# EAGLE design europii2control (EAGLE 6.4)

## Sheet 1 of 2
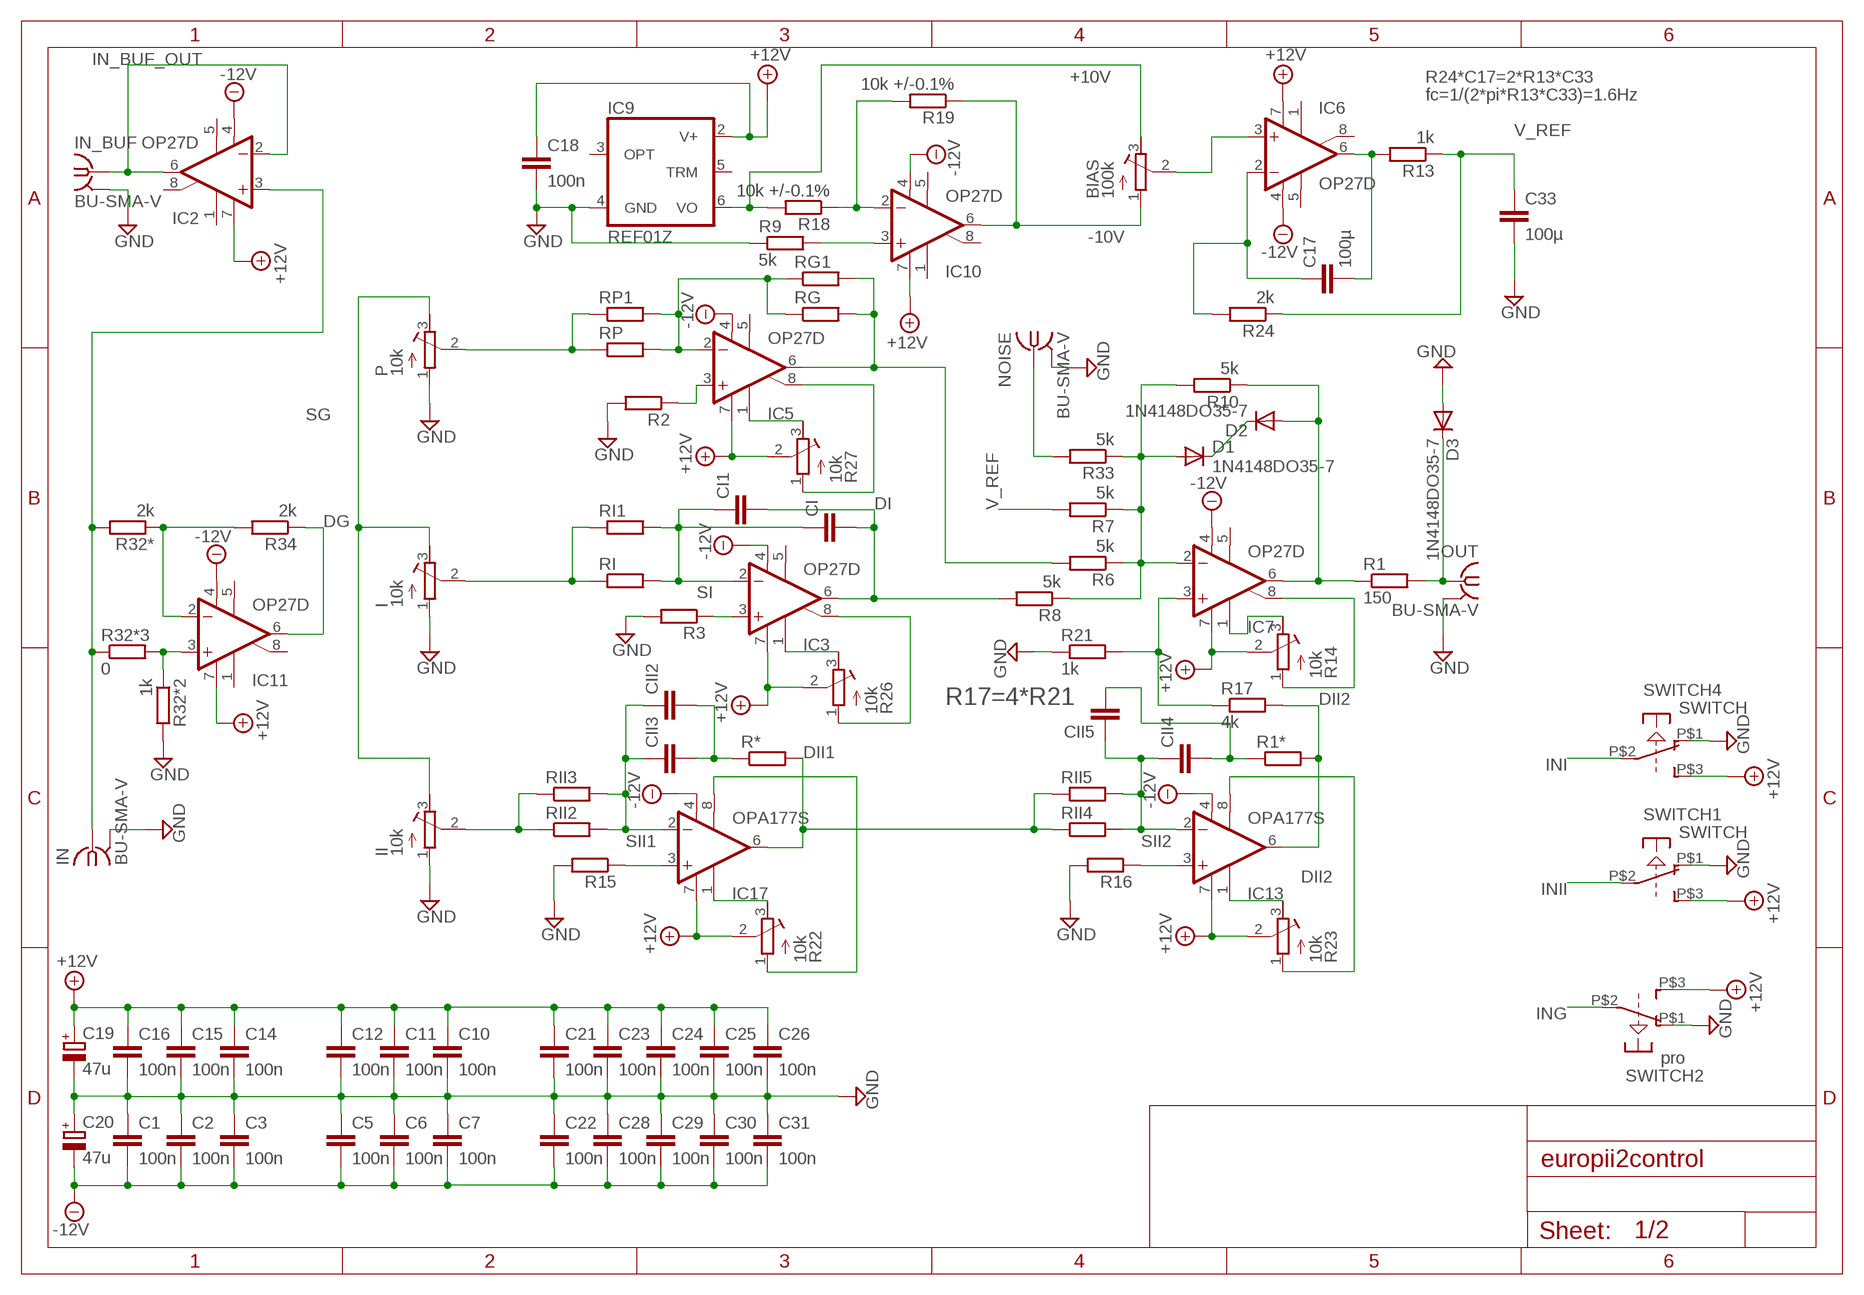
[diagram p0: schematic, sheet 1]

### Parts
BIAS  100k  R-TRIMM64X  [RTRIM64X]
C1  100n  C-EUC0805  [C0805]
C2  100n  C-EUC0805  [C0805]
C3  100n  C-EUC0805  [C0805]
C5  100n  C-EUC0805  [C0805]
C6  100n  C-EUC0805  [C0805]
C7  100n  C-EUC0805  [C0805]
C10  100n  C-EUC0805  [C0805]
C11  100n  C-EUC0805  [C0805]
C12  100n  C-EUC0805  [C0805]
C14  100n  C-EUC0805  [C0805]
C15  100n  C-EUC0805  [C0805]
C16  100n  C-EUC0805  [C0805]
C17  100µ  C-EUC1210K  [C1210K]
C18  100n  C-EUC0805  [C0805]
C19  47u  CPOL-EUCT7343  [CT7343]
C20  47u  CPOL-EUCT7343  [CT7343]
C21  100n  C-EUC0805  [C0805]
C22  100n  C-EUC0805  [C0805]
C23  100n  C-EUC0805  [C0805]
C24  100n  C-EUC0805  [C0805]
C25  100n  C-EUC0805  [C0805]
C26  100n  C-EUC0805  [C0805]
C28  100n  C-EUC0805  [C0805]
C29  100n  C-EUC0805  [C0805]
C30  100n  C-EUC0805  [C0805]
C31  100n  C-EUC0805  [C0805]
C33  100µ  C-EUC1210K  [C1210K]
CI  C-EUC1210  [C1210]
CI1  C-EU050-025X075  [C050-025X075]
CII2  C-EU050-025X075  [C050-025X075]
CII3  C-EUC1210  [C1210]
CII4  C-EUC1210  [C1210]
CII5  C-EU050-025X075  [C050-025X075]
D1  1N4148DO35-7  [DO35-7]
D2  1N4148DO35-7  [DO35-7]
D3  1N4148DO35-7  [DO35-7]
I  10k  R-TRIMM64X  [RTRIM64X]
IC2  OP27D  [SO08]
IC3  OP27D  [SO08]
IC5  OP27D  [SO08]
IC6  OP27D  [SO08]
IC7  OP27D  [SO08]
IC9  REF01Z  [DIL08]
IC10  OP27D  [SO08]
IC11  OP27D  [SO08]
IC13  OPA177S  [SO08]
IC17  OPA177S  [SO08]
II  10k  R-TRIMM64X  [RTRIM64X]
IN  BU-SMA-V  [BU-SMA-V]
IN_BUF  BU-SMA-V  [BU-SMA-V]
NOISE  BU-SMA-V  [BU-SMA-V]
OUT  BU-SMA-V  [BU-SMA-V]
P  10k  R-TRIMM64X  [RTRIM64X]
R1  150  R-EU_R0805  [R0805]
R1*  R-EU_R0805  [R0805]
R2  R-EU_R0805  [R0805]
R3  R-EU_R0805  [R0805]
R6  5k  R-EU_R0805  [R0805]
R7  5k  R-EU_R0805  [R0805]
R8  5k  R-EU_R0805  [R0805]
R9  5k  R-EU_R0805  [R0805]
R10  5k  R-EU_R0805  [R0805]
R13  1k  R-EU_R0805  [R0805]
R14  10k  R-TRIMM3224W  [RTRIM3224W]
R15  R-EU_R0805  [R0805]
R16  R-EU_R0805  [R0805]
R17  4k  R-EU_R0805  [R0805]
R18  10k +/-0.1%  R-EU_R0805  [R0805]
R19  10k +/-0.1%  R-EU_R0805  [R0805]
R21  1k  R-EU_R0805  [R0805]
R22  10k  R-TRIMM3224W  [RTRIM3224W]
R23  10k  R-TRIMM3224W  [RTRIM3224W]
R24  2k  R-EU_R0805  [R0805]
R26  10k  R-TRIMM3224W  [RTRIM3224W]
R27  10k  R-TRIMM3224W  [RTRIM3224W]
R32*  2k  R-EU_R0805  [R0805]
R32*2  1k  R-EU_R0805  [R0805]
R32*3  0  R-EU_R0805  [R0805]
R33  5k  R-EU_R0805  [R0805]
R34  2k  R-EU_R0805  [R0805]
R*  R-EU_R0805  [R0805]
RG  R-EU_R0805  [R0805]
RG1  R-EU_0207/12  [0207/12]
RI  R-EU_R0805  [R0805]
RI1  R-EU_0207/12  [0207/12]
RII2  R-EU_R0805  [R0805]
RII3  R-EU_0207/12  [0207/12]
RII4  R-EU_R0805  [R0805]
RII5  R-EU_0207/12  [0207/12]
RP  R-EU_R0805  [R0805]
RP1  R-EU_0207/12  [0207/12]
SWITCH1  SWITCH  [SWITCH]
SWITCH2  pro  SWITCH  [SWITCH]
SWITCH4  SWITCH  [SWITCH]

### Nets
+10V: BIAS.3(A) IC9.6(VO) R18.2 ; also sheet 2
+12V: C10.1 C11.1 C12.1 C14.1 C15.1 C16.1 C18.1 C19.+ C21.1 C23.1 C24.1 C25.1 C26.1 IC2.7(V+) IC3.7(V+) IC5.7(V+) IC6.7(V+) IC7.7(V+) IC9.2(V+) IC10.7(V+) IC11.7(V+) IC13.7(V+) IC17.7(V+) R14.2(S) R22.2(S) R23.2(S) R26.2(S) R27.2(S) SWITCH1.P$3(S) SWITCH2.P$3(S) SWITCH4.P$3(S) ; also sheet 2
-10V: BIAS.1(E) IC10.6(OUT) R19.1 ; also sheet 2
-12V: C1.2 C2.2 C3.2 C5.2 C6.2 C7.2 C20.- C22.2 C28.2 C29.2 C30.2 C31.2 IC2.4(V-) IC3.4(V-) IC5.4(V-) IC6.4(V-) IC7.4(V-) IC10.4(V-) IC11.4(V-) IC13.4(V-) IC17.4(V-) ; also sheet 2
DG: IC11.6(OUT) R34.1 ; also sheet 2
DI: CI1.2 CI.2 IC3.6(OUT) R8.2 ; also sheet 2
DII1: IC17.6(OUT) R*.2 RII4.1 RII5.1 ; also sheet 2
DII2: IC13.6(OUT) R1*.2 R17.2 ; also sheet 2
ERR_BUF: D2.A IC7.6(OUT) R1.1 R10.1 ; also sheet 2
GND: C1.1 C2.1 C3.1 C5.1 C6.1 C7.1 C10.2 C11.2 C12.2 C14.2 C15.2 C16.2 C18.2 C19.- C20.+ C21.2 C22.1 C23.2 C24.2 C25.2 C26.2 C28.1 C29.1 C30.1 C31.1 C33.2 D3.A I.1(E) IC9.4(GND) II.1(E) IN.2(GND) IN_BUF.2(GND) NOISE.2(GND) OUT.2(GND) P.1(E) R2.2 R3.2 R9.1 R15.2 R16.2 R21.1 R32*2.2 SWITCH1.P$1(O) SWITCH2.P$1(O) SWITCH4.P$1(O) ; also sheet 2
IN_BUF_OUT: IC2.2(-IN) IC2.6(OUT) IN_BUF.1 ; also sheet 2
ING: SWITCH2.P$2(P) ; also sheet 2
INI: SWITCH4.P$2(P) ; also sheet 2
INII: SWITCH1.P$2(P) ; also sheet 2
N$1: IC10.3(+IN) R9.2
N$3: IC3.8(ON2) R26.1(E)
N$4: IC10.2(-IN) R18.1 R19.2
N$5: D1.A IC7.2(-IN) R6.1 R7.1 R8.1 R10.2 R33.1
N$9: IC5.2(-IN) RG1.1 RG.1 RP1.2 RP.2
N$10: IC13.1(TRIM1) R23.3(A)
N$11: II.2(S) RII2.1 RII3.1
N$13: D3.C OUT.1 R1.2
N$15: C17.2 IC6.6(OUT) R13.2
N$17: IC5.3(+IN) R2.1
N$18: IC3.3(+IN) R3.1
N$19: P.2(S) RP1.1 RP.1
N$21: IC11.3(+IN) R32*2.1 R32*3.2
N$24: IC17.3(+IN) R15.1
N$25: IC13.3(+IN) R16.1
N$26: IC7.3(+IN) R17.1 R21.2
N$27: IC7.1(ON1) R14.3(A)
N$28: IC7.8(ON2) R14.1(E)
N$29: IC3.1(ON1) R26.3(A)
N$30: I.2(S) RI1.1 RI.1
N$31: IC17.1(TRIM1) R22.3(A)
N$32: IC5.8(ON2) R27.1(E)
N$33: IC5.1(ON1) R27.3(A)
N$34: IC17.8(TRIM2) R22.1(E)
N$37: IC5.6(OUT) R6.2 RG1.2 RG.2
N$39: D1.C D2.C
N$40: CII2.2 CII3.2 R*.1
N$41: IC11.2(-IN) R32*.1 R34.2
N$42: CII4.2 CII5.2 R1*.1
N$43: IC2.3(+IN) IN.1 R32*3.1 R32*.2
N$46: IC13.8(TRIM2) R23.1(E)
N$47: NOISE.1 R33.2
N$50: C17.1 IC6.2(-IN) R24.2
N$51: BIAS.2(S) IC6.3(+IN)
SG: I.3(A) II.3(A) P.3(A) ; also sheet 2
SI: CI1.1 CI.1 IC3.2(-IN) RI1.2 RI.2 ; also sheet 2
SII1: CII2.1 CII3.1 IC17.2(-IN) RII2.2 RII3.2 ; also sheet 2
SII2: CII4.1 CII5.1 IC13.2(-IN) RII4.2 RII5.2 ; also sheet 2
V_REF: C33.1 R7.2 R13.1 R24.1
Unconnected: IC2.1(ON1) IC2.5(OPT) IC2.8(ON2) IC3.5(OPT) IC5.5(OPT) IC6.1(ON1) IC6.5(OPT) IC6.8(ON2) IC7.5(OPT) IC9.3(OPT) IC9.5(TRM) IC10.1(ON1) IC10.5(OPT) IC10.8(ON2) IC11.1(ON1) IC11.5(OPT) IC11.8(ON2)

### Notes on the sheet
- R24*C17=2*R13*C33
- fc=1/(2*pi*R13*C33)=1.6Hz
- R17=4*R21

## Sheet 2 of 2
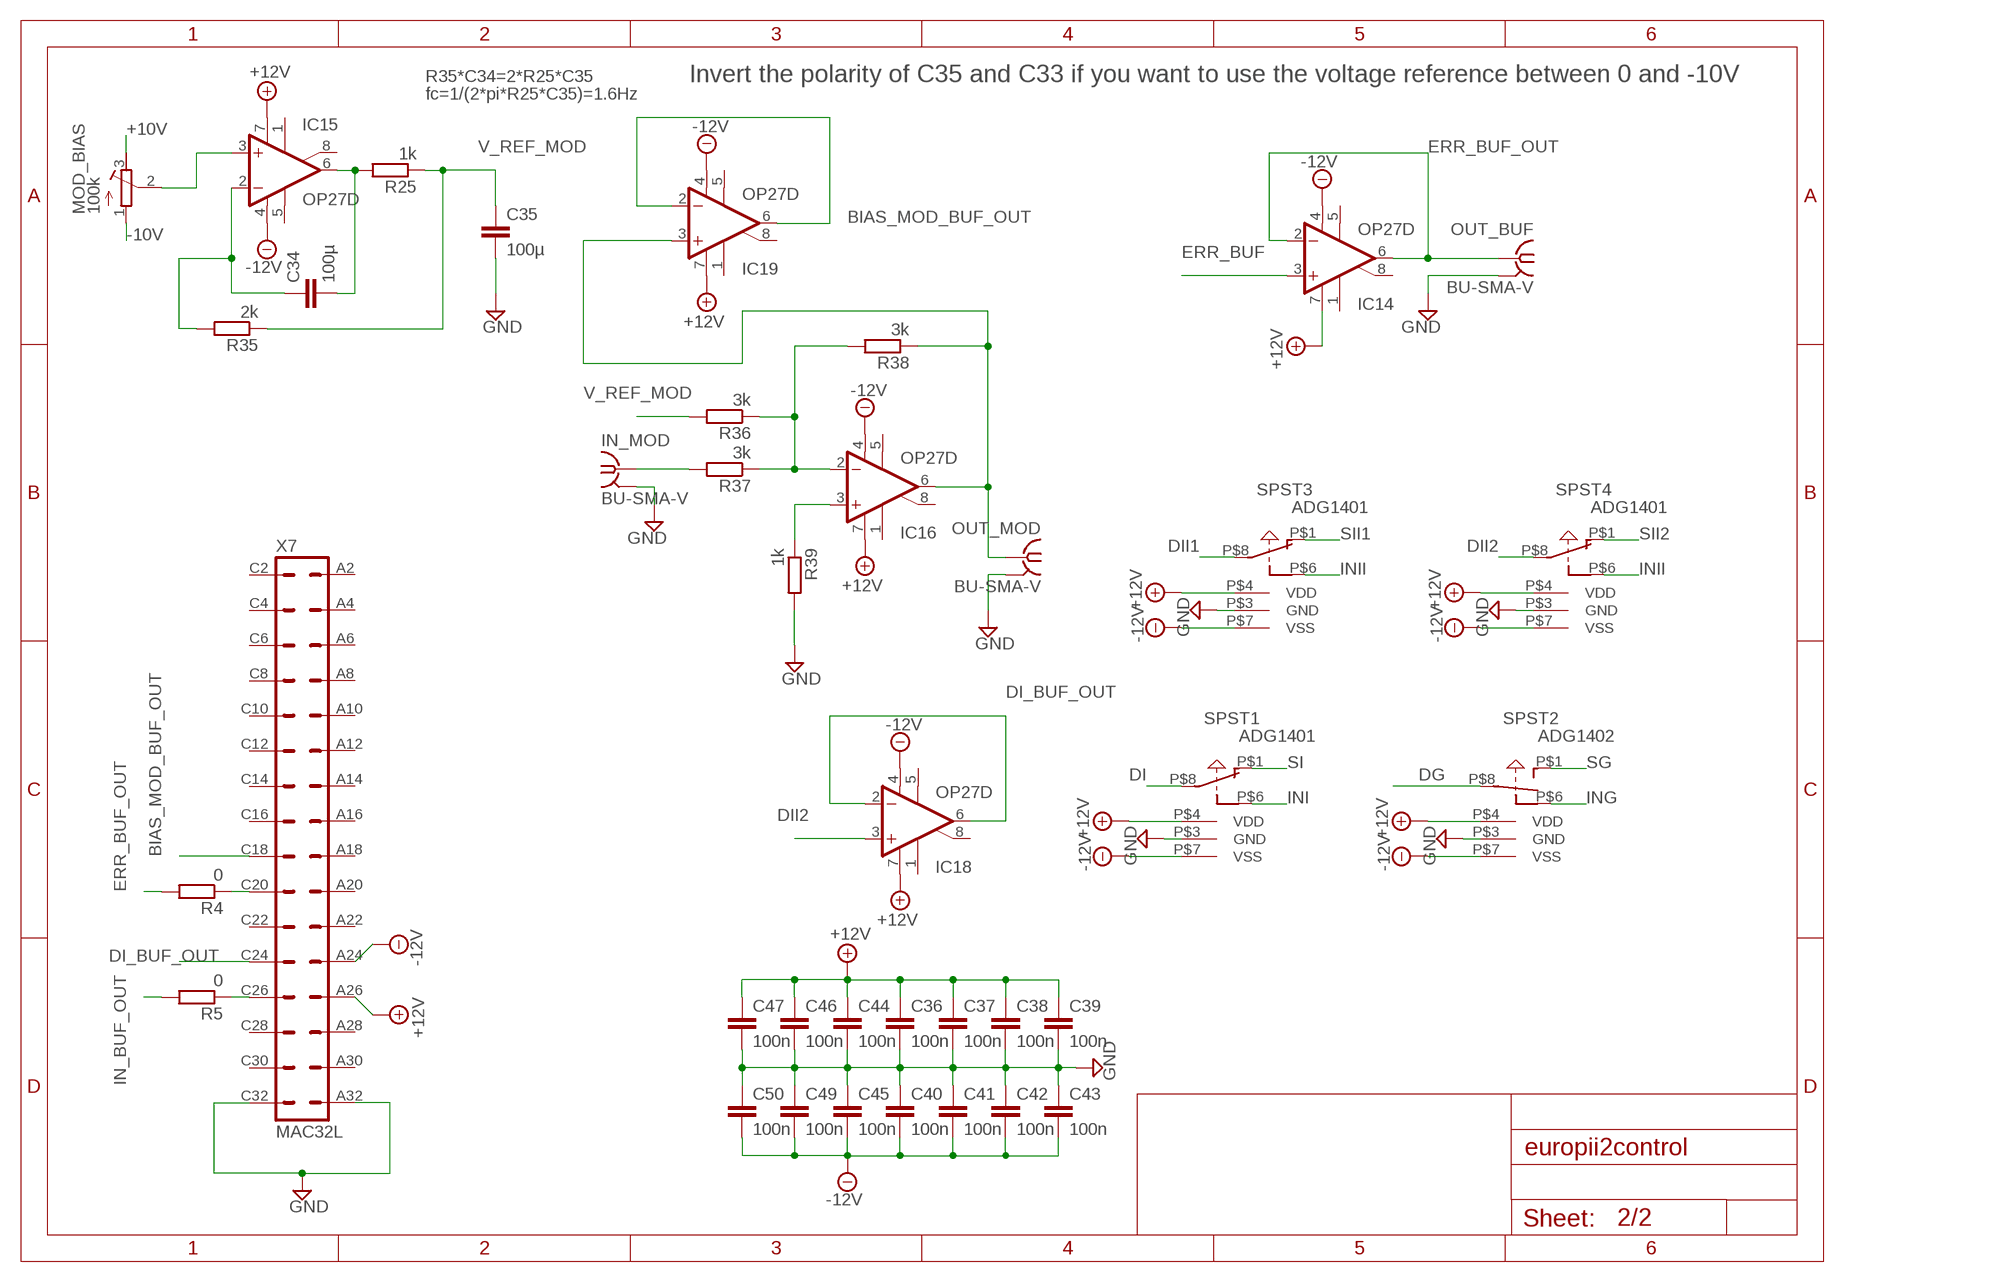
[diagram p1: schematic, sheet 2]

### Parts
C34  100µ  C-EUC1210K  [C1210K]
C35  100µ  C-EUC1210K  [C1210K]
C36  100n  C-EUC0805  [C0805]
C37  100n  C-EUC0805  [C0805]
C38  100n  C-EUC0805  [C0805]
C39  100n  C-EUC0805  [C0805]
C40  100n  C-EUC0805  [C0805]
C41  100n  C-EUC0805  [C0805]
C42  100n  C-EUC0805  [C0805]
C43  100n  C-EUC0805  [C0805]
C44  100n  C-EUC0805  [C0805]
C45  100n  C-EUC0805  [C0805]
C46  100n  C-EUC0805  [C0805]
C47  100n  C-EUC0805  [C0805]
C49  100n  C-EUC0805  [C0805]
C50  100n  C-EUC0805  [C0805]
IC14  OP27D  [SO08]
IC15  OP27D  [SO08]
IC16  OP27D  [SO08]
IC18  OP27D  [SO08]
IC19  OP27D  [SO08]
IN_MOD  BU-SMA-V  [BU-SMA-V]
MOD_BIAS  100k  R-TRIMM64X  [RTRIM64X]
OUT_BUF  BU-SMA-V  [BU-SMA-V]
OUT_MOD  BU-SMA-V  [BU-SMA-V]
R4  0  R-EU_R0805  [R0805]
R5  0  R-EU_R0805  [R0805]
R25  1k  R-EU_R0805  [R0805]
R35  2k  R-EU_R0805  [R0805]
R36  3k  R-EU_R0805  [R0805]
R37  3k  R-EU_R0805  [R0805]
R38  3k  R-EU_R0805  [R0805]
R39  1k  R-EU_R0805  [R0805]
SPST1  ADG1401  [MSOP-RM8]
SPST2  ADG1402  [MSOP-RM8]
SPST3  ADG1401  [MSOP-RM8]
SPST4  ADG1401  [MSOP-RM8]
X7  MAC32L  [MAC32L]

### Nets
+10V: MOD_BIAS.3(A) ; also sheet 1
+12V: C36.1 C37.1 C38.1 C39.1 C44.1 C46.1 C47.1 IC14.7(V+) IC15.7(V+) IC16.7(V+) IC18.7(V+) IC19.7(V+) SPST1.P$4(VDD) SPST2.P$4(VDD) SPST3.P$4(VDD) SPST4.P$4(VDD) X7.A26 ; also sheet 1
-10V: MOD_BIAS.1(E) ; also sheet 1
-12V: C40.2 C41.2 C42.2 C43.2 C45.2 C49.2 C50.2 IC14.4(V-) IC15.4(V-) IC16.4(V-) IC18.4(V-) IC19.4(V-) SPST1.P$7(VSS) SPST2.P$7(VSS) SPST3.P$7(VSS) SPST4.P$7(VSS) X7.A24 ; also sheet 1
BIAS_MOD_BUF_OUT: IC19.2(-IN) IC19.6(OUT) X7.C18
DG: SPST2.P$8(D) ; also sheet 1
DI: SPST1.P$8(D) ; also sheet 1
DI_BUF_OUT: IC18.2(-IN) IC18.6(OUT) X7.C24
DII1: SPST3.P$8(D) ; also sheet 1
DII2: IC18.3(+IN) SPST4.P$8(D) ; also sheet 1
ERR_BUF: IC14.3(+IN) ; also sheet 1
ERR_BUF_OUT: IC14.2(-IN) IC14.6(OUT) OUT_BUF.1 R4.2
GND: C35.2 C36.2 C37.2 C38.2 C39.2 C40.1 C41.1 C42.1 C43.1 C44.2 C45.1 C46.2 C47.2 C49.1 C50.1 IN_MOD.2(GND) OUT_BUF.2(GND) OUT_MOD.2(GND) R39.2 SPST1.P$3(GND) SPST2.P$3(GND) SPST3.P$3(GND) SPST4.P$3(GND) X7.A32 X7.C32 ; also sheet 1
IN_BUF_OUT: R5.2 ; also sheet 1
ING: SPST2.P$6(IN) ; also sheet 1
INI: SPST1.P$6(IN) ; also sheet 1
INII: SPST3.P$6(IN) SPST4.P$6(IN) ; also sheet 1
N$6: R4.1 X7.C20
N$7: IC16.3(+IN) R39.1
N$8: IN_MOD.1 R37.2
N$16: IC16.2(-IN) R36.1 R37.1 R38.2
N$20: IC16.6(OUT) IC19.3(+IN) OUT_MOD.1 R38.1
N$38: R5.1 X7.C26
N$52: C34.2 IC15.6(OUT) R25.2
N$53: C34.1 IC15.2(-IN) R35.2
N$54: IC15.3(+IN) MOD_BIAS.2(S)
SG: SPST2.P$1(S) ; also sheet 1
SI: SPST1.P$1(S) ; also sheet 1
SII1: SPST3.P$1(S) ; also sheet 1
SII2: SPST4.P$1(S) ; also sheet 1
V_REF_MOD: C35.1 R25.1 R35.1 R36.2
Unconnected: IC14.1(ON1) IC14.5(OPT) IC14.8(ON2) IC15.1(ON1) IC15.5(OPT) IC15.8(ON2) IC16.1(ON1) IC16.5(OPT) IC16.8(ON2) IC18.1(ON1) IC18.5(OPT) IC18.8(ON2) IC19.1(ON1) IC19.5(OPT) IC19.8(ON2) X7.A2 X7.A4 X7.A6 X7.A8 X7.A10 X7.A12 X7.A14 X7.A16 X7.A18 X7.A20 X7.A22 X7.A28 X7.A30 X7.C2 X7.C4 X7.C6 X7.C8 X7.C10 X7.C12 X7.C14 X7.C16 X7.C22 X7.C28 X7.C30

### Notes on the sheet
- R35*C34=2*R25*C35 | Invert the polarity of C35 and C33 if you want to use the voltage reference between 0 and -10V
- fc=1/(2*pi*R25*C35)=1.6Hz

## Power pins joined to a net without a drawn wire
GND: IN.3(GND) IN.4(GND) IN.5(GND) IN_BUF.3(GND) IN_BUF.4(GND) IN_BUF.5(GND) IN_MOD.3(GND) IN_MOD.4(GND) IN_MOD.5(GND) NOISE.3(GND) NOISE.4(GND) NOISE.5(GND) OUT.3(GND) OUT.4(GND) OUT.5(GND) OUT_BUF.3(GND) OUT_BUF.4(GND) OUT_BUF.5(GND) OUT_MOD.3(GND) OUT_MOD.4(GND) OUT_MOD.5(GND)

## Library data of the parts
BIAS I II MOD_BIAS P R14 R22 R23 R26 R27 = rcl:R-TRIMM: Trimm resistor
C1-C3 C5-C7 C10-C12 C14-C18 C21-C26 C28-C31 C33-C47 C49 C50 CI CI1 CII2-CII5 = rcl:C-EU: CAPACITOR, European symbol
C19 C20 = rcl:CPOL-EU: POLARIZED CAPACITOR, European symbol
D1-D3 = diode:1N4148: DIODE
IC2 IC3 IC5-IC7 IC10 IC11 IC14-IC16 IC18 IC19 = linear:OP27: OP AMP
IC9 = linear:REF01: VOLTAGE REFERENCE
IC13 IC17 = burr-brown:OPA177: Precision Operational Amplifier
IN IN_BUF IN_MOD NOISE OUT OUT_BUF OUT_MOD = con-coax:BU-SMA-V: FEMALE SMA CONNECTOR Radiall distributor RS 112-3794
R1 R1* R2-R10 R13 R15-R19 R21 R24 R25 R32* R32*2 R32*3 R33-R39 R* RG RG1 RI RI1 RII2-RII5 RP RP1 = rcl:R-EU_: RESISTOR, European symbol
SPST1 SPST3 SPST4 = srinos-lib:ADG1401
SPST2 = srinos-lib:ADG1402
SWITCH1 SWITCH2 SWITCH4 = srinos-lib:SWITCH
X7 = con-vg:MAC32L: CONNECTOR male, 32 pins, block, type D, rows AC, grid 5.08 mm with mounting clip

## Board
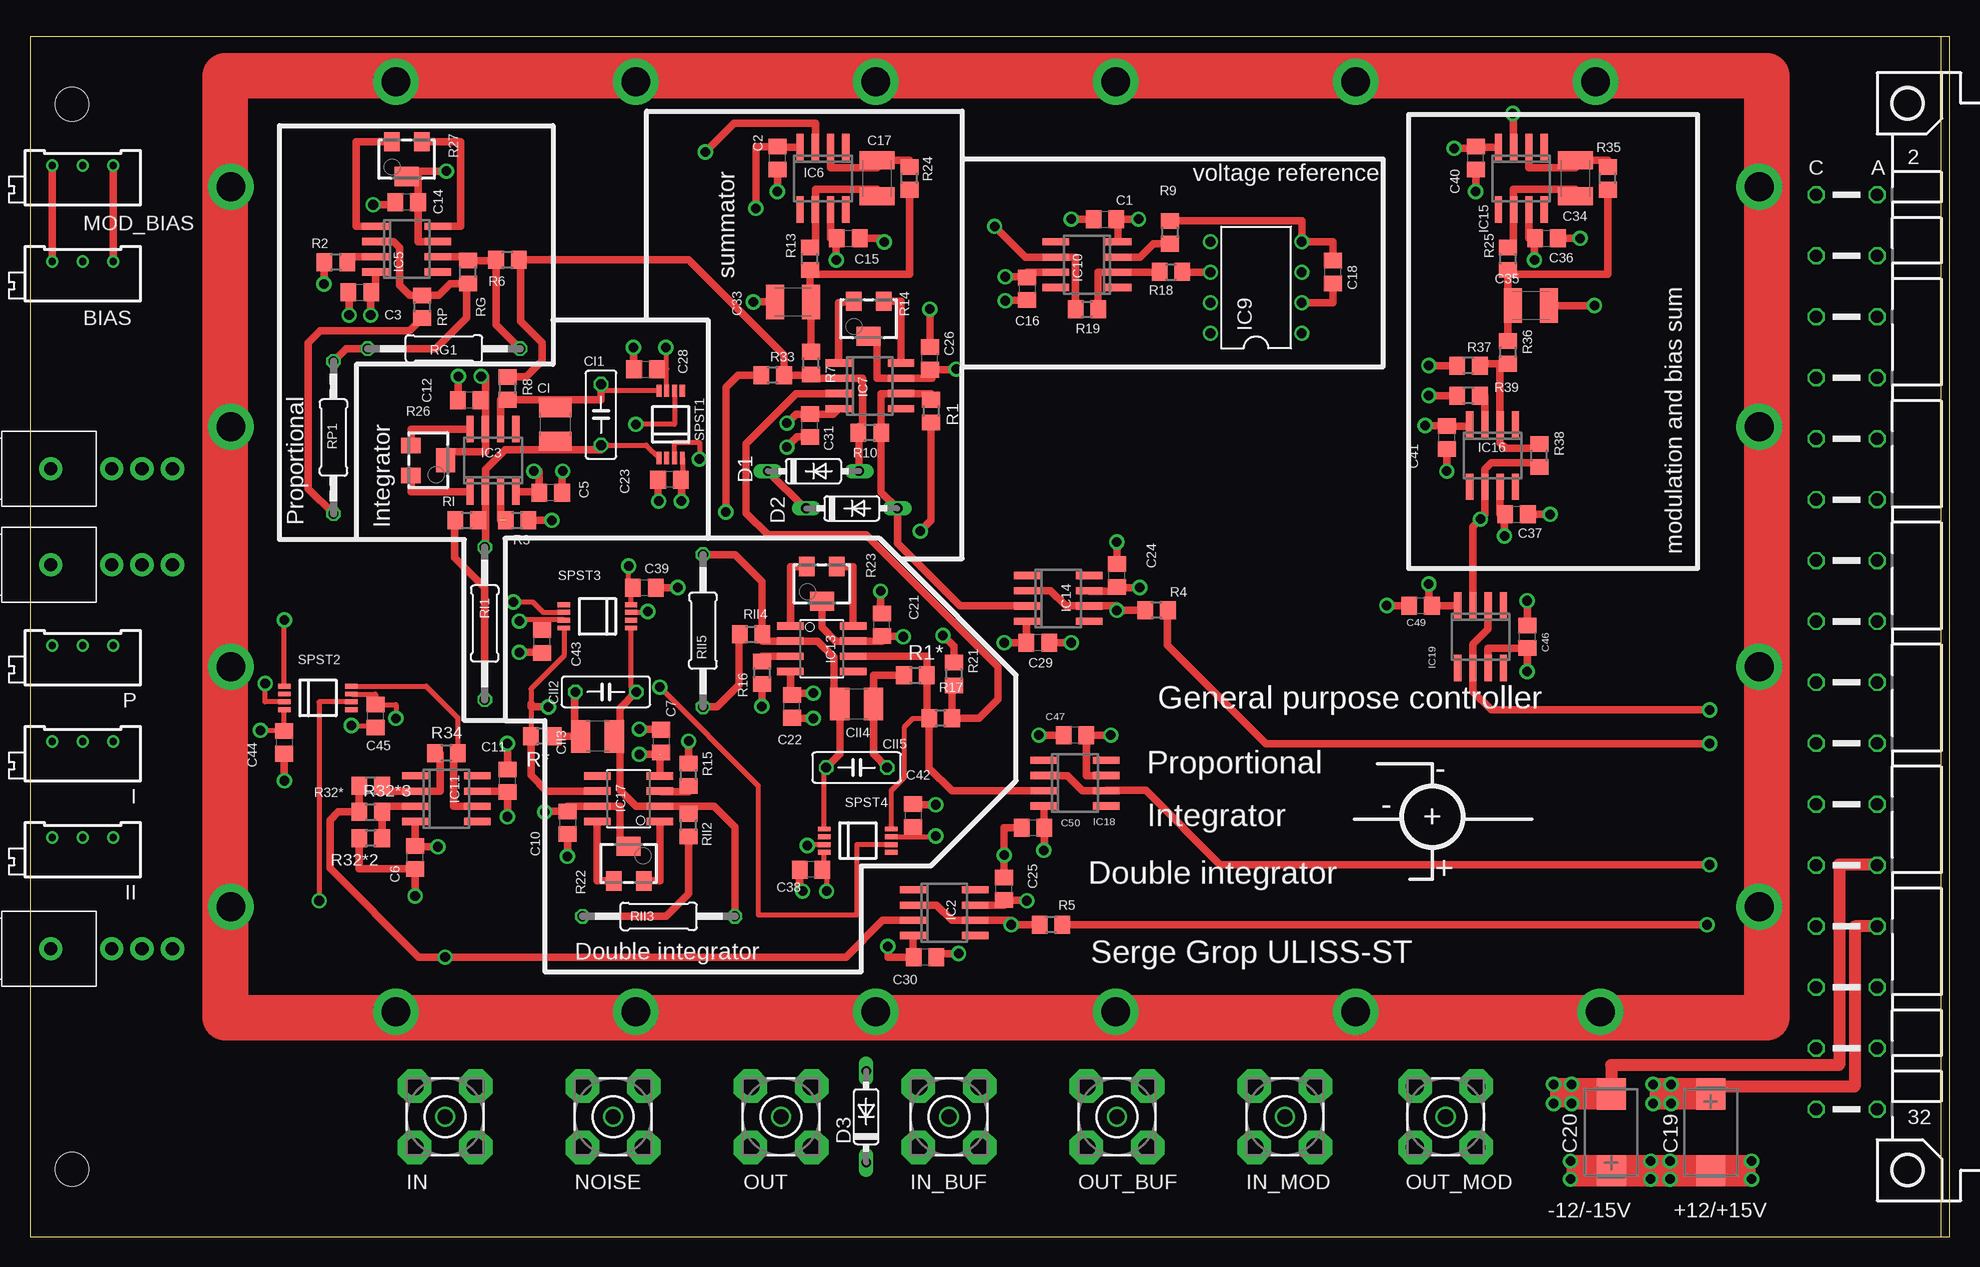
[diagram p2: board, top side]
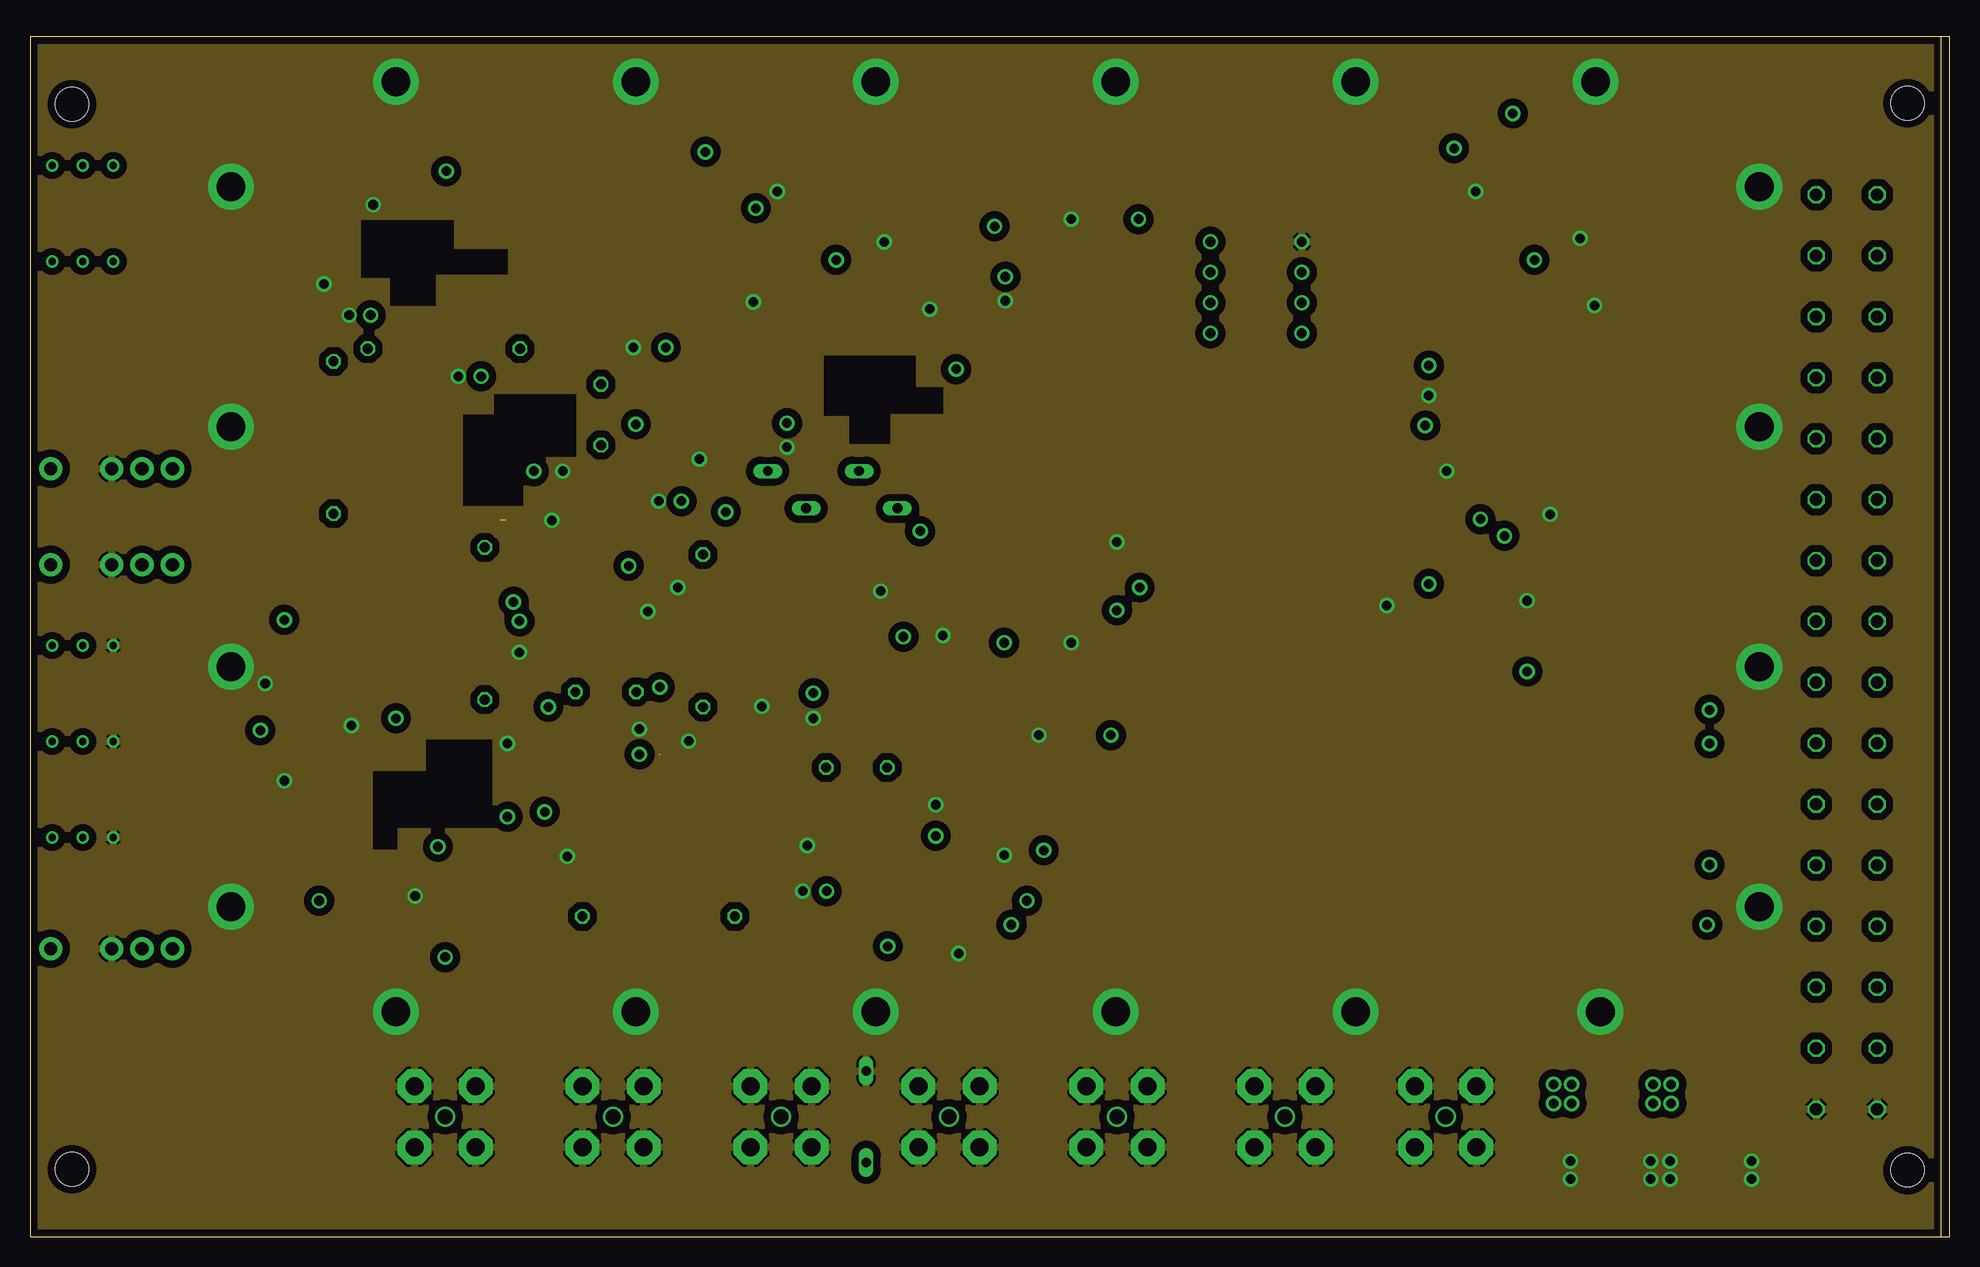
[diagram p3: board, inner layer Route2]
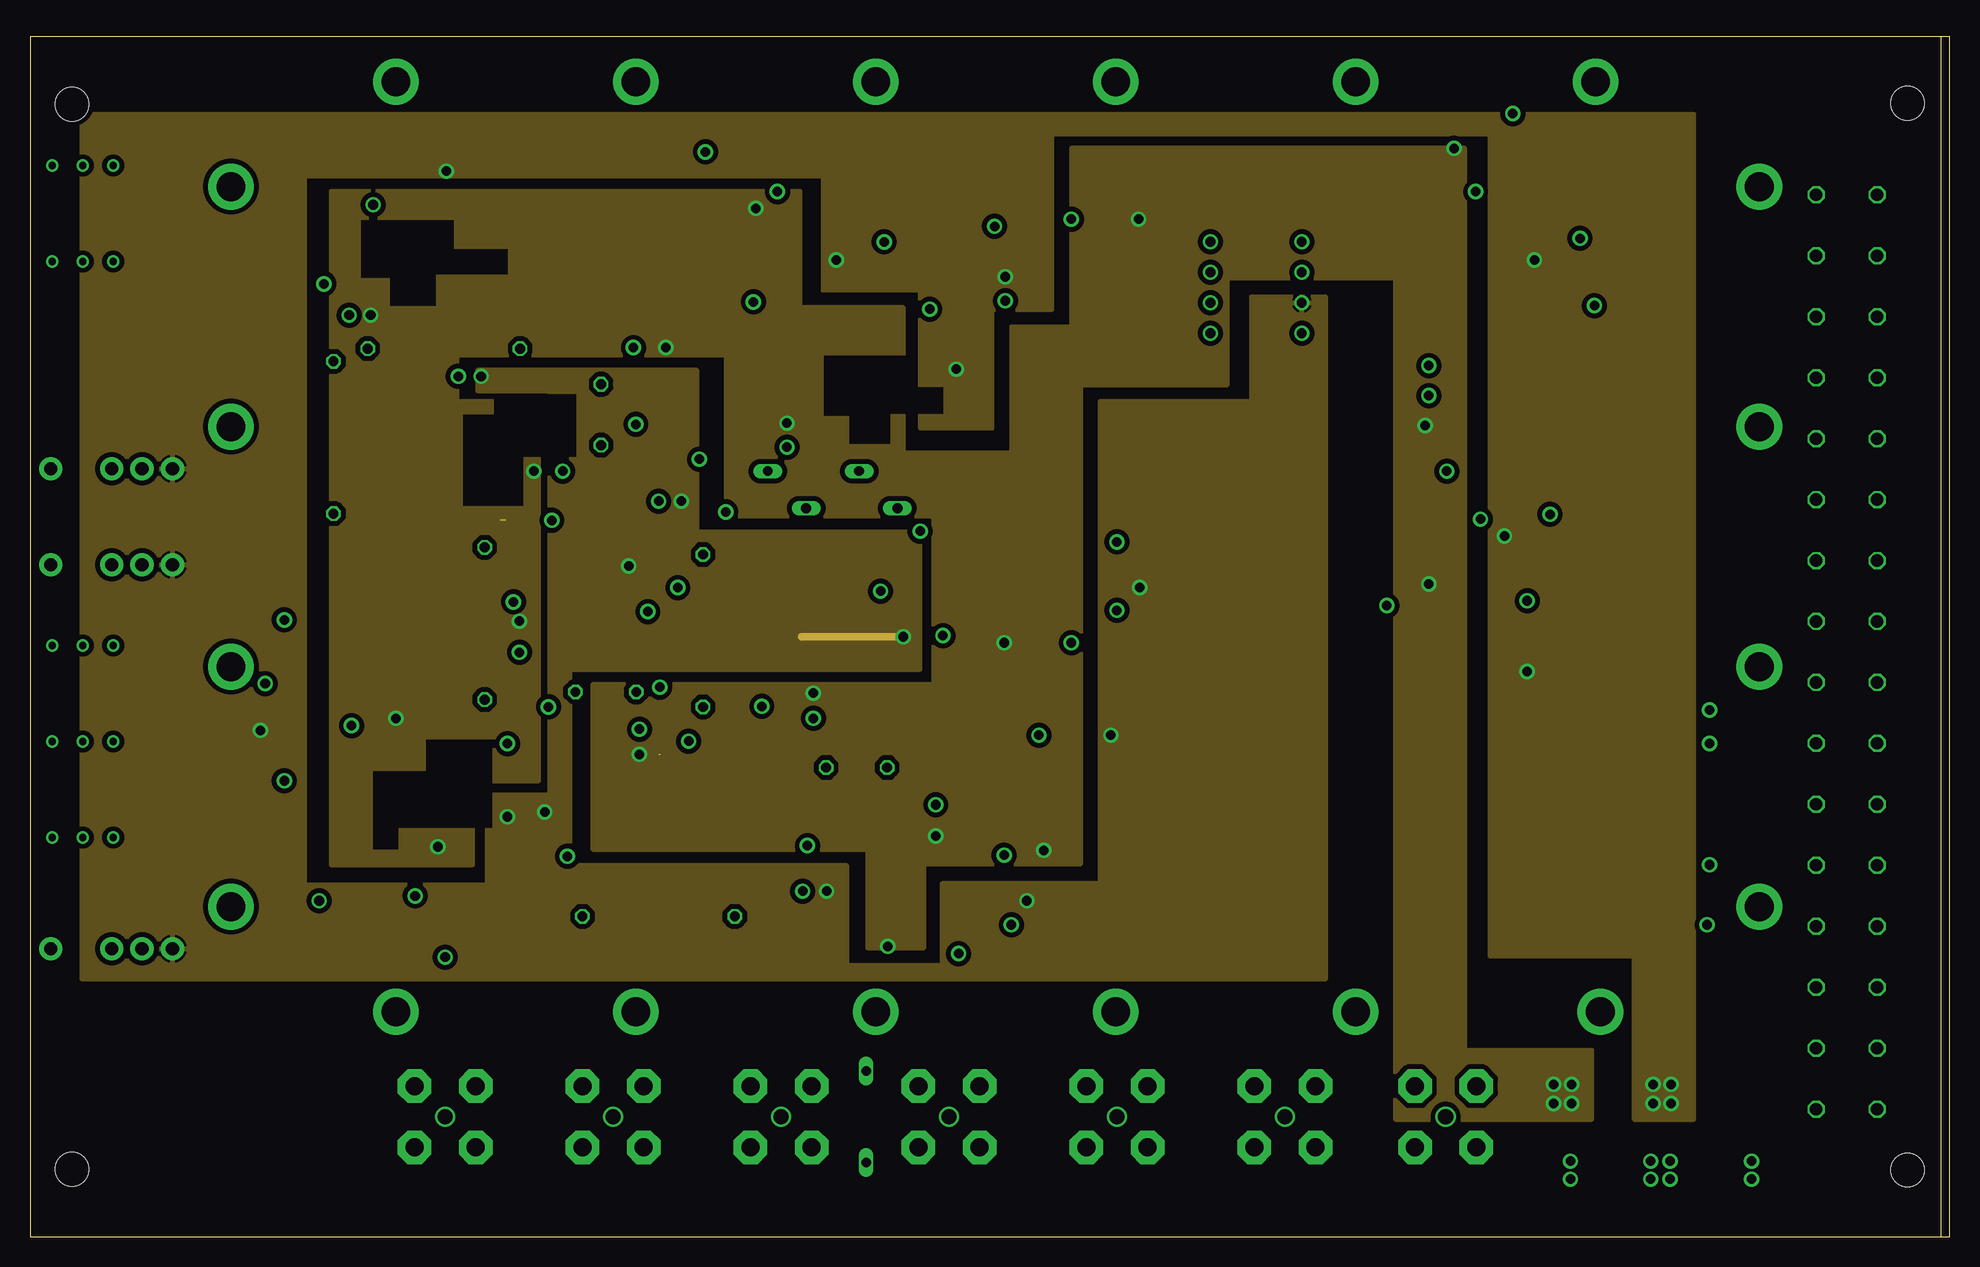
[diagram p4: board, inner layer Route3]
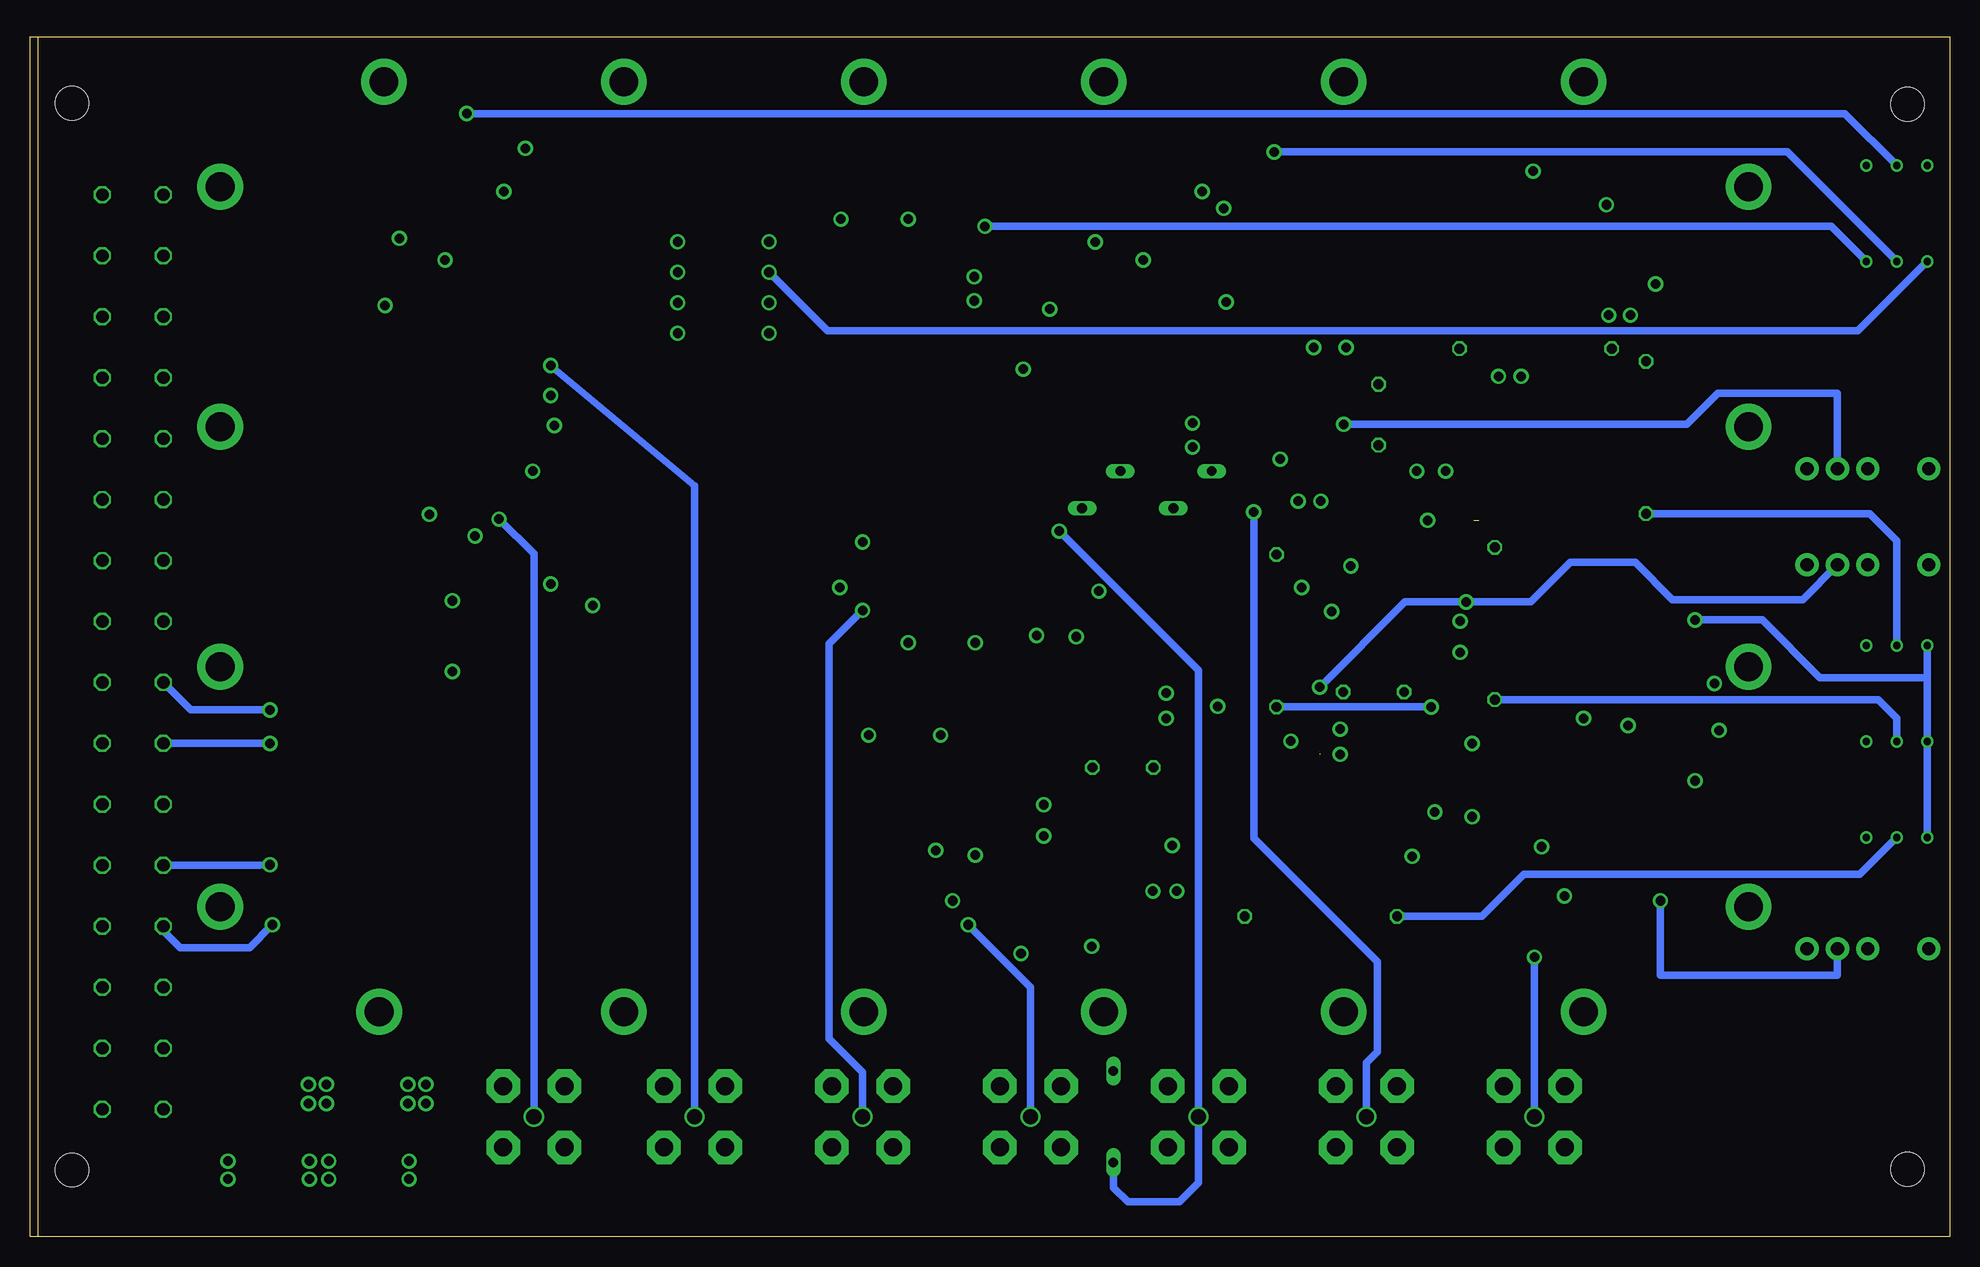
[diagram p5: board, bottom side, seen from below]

Size 160 x 100.03 mm. Coordinates in mm from the lower left corner, seen from the top.
Outline: 0,0.01 160,0.01 160,100.01 0,100.01 0,0.01
Copper layers (1*2*3*16): Top 0.035mm / dielectric 0.38mm / Route2 0.035mm / dielectric 0.71mm / Route3 0.035mm / dielectric 0.38mm / Bottom 0.035mm
Design rules "PCB-POOL-Standard-4-layers": minimum track width 0.15mm, minimum drill 0.3mm, track to track 0.15mm, track to pad 0.15mm, pad to pad 0.15mm, via to via 0.15mm, smd to smd 0.15mm, copper to edge 0.3mm, drill to drill 0.2mm, minimum pad ring 0.2mm, minimum via ring 0.15mm, stop-mask expansion 0.075mm, vias tented up to drill 0mil, thermal gap 0.2mm
Holes 2.8 mm at 3.5,5.64 3.5,94.39

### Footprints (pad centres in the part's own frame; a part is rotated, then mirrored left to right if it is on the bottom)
RTRIM64X = drill 0.61: 1 1.27,-2.54; 2 1.27,0; 3 1.27,2.54
C0805 = smd 1.3 x 1.5: 1 -0.95,0; 2 0.95,0
C1210K = smd 1.5 x 2.9: 1 -1.5,0; 2 1.5,0
CT7343 = smd 2.6 x 2.4: + -3.2,0; - 3.2,0
C1210 = smd 1.6 x 2.7: 1 -1.4,0; 2 1.4,0
C050-025X075 = drill 0.813 octagon: 1 -2.54,0; 2 2.54,0
DO35-7 = drill 0.813 long: A 3.81,0; C -3.81,0
SO08 = smd 0.6 x 2.2: 1 -1.905,-2.6; 2 -0.635,-2.6; 3 0.635,-2.6; 4 1.905,-2.6; 5 1.905,2.6; 6 0.635,2.6; 7 -0.635,2.6; 8 -1.905,2.6
DIL08 = drill 0.813 pad 1.27: 1 -3.81,-3.81; 2 -1.27,-3.81; 3 1.27,-3.81; 4 3.81,-3.81; 5 3.81,3.81; 6 1.27,3.81; 7 -1.27,3.81; 8 -3.81,3.81
SO08' = smd 0.61 x 2.21: 1 -1.905,-2.616; 2 -0.635,-2.616; 3 0.635,-2.616; 4 1.905,-2.616; 5 1.905,2.616; 6 0.635,2.616; 7 -0.635,2.616; 8 -1.905,2.616
BU-SMA-V = drill 1.27: 1 0,0 | drill 1.5 pad 2.794 octagon: 2 -2.55,2.55; 3 2.55,2.55; 4 2.55,-2.55; 5 -2.55,-2.55
R0805 = smd 1.3 x 1.5: 1 -0.95,0; 2 0.95,0
RTRIM3224W = smd 1.3 x 1.6: 1 -1.25,-1.45; 3 1.25,-1.45 | smd 2 x 1.6: 2 0,1.45
0207/12 = drill 0.813 octagon: 1 -6.35,0; 2 6.35,0
MSOP-RM8 = smd 0.41 x 1.02: P$1 -0.975,-2.8; P$2 -0.325,-2.8; P$3 0.325,-2.8; P$4 0.975,-2.8; P$6 0.325,2.8; P$7 -0.325,2.8; P$8 -0.975,2.8 | smd 0.42 x 1.02: P$5 0.975,2.8
SWITCH = drill 1.1 pad 1.93: P$1 0,0; P$2 0,2.54; P$3 0,5.08; P$4 0,-5.08
MAC32L = drill 1.016 octagon: A2 -2.54,36.83; A4 -2.54,31.75; A6 -2.54,26.67; A8 -2.54,21.59; A10 -2.54,16.51; A12 -2.54,11.43; A14 -2.54,6.35; A16 -2.54,1.27; A18 -2.54,-3.81; A20 -2.54,-8.89; A22 -2.54,-13.97; A24 -2.54,-19.05; A26 -2.54,-24.13; A28 -2.54,-29.21; A30 -2.54,-34.29; A32 -2.54,-39.37; C2 -7.62,36.83; C4 -7.62,31.75; C6 -7.62,26.67; C8 -7.62,21.59; C10 -7.62,16.51; C12 -7.62,11.43; C14 -7.62,6.35; C16 -7.62,1.27; C18 -7.62,-3.81; C20 -7.62,-8.89; C22 -7.62,-13.97; C24 -7.62,-19.05; C26 -7.62,-24.13; C28 -7.62,-29.21; C30 -7.62,-34.29; C32 -7.62,-39.37 | hole 2.794: 0,44.45; 0,-44.45

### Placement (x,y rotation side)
BIAS  4.4,80.01 90 top
C1  89.6,84.81 0 top
C2  62.3,89.91 90 top
C3  27.5,78.71 0 top
C5  43.4,62.01 180 top
C6  32.1,31.61 90 top
C7  52.6,41.31 270 top
C10  44.8,34.51 270 top
C11  39.8,38.01 90 top
C12  36.6,69.71 180 top
C14  31.4,86.21 180 top
C15  68.2,83.21 0 top
C16  83.1,79.01 270 top
C17  70.6,88.21 270 top
C18  108.6,80.41 90 top
C19  140.1,8.71 270 top
C20  131.8,8.71 90 top
C21  71,51.01 90 top
C22  63.5,44.21 90 top
C23  53.3,63.11 180 top
C24  90.6,55.11 90 top
C25  81.2,29.01 90 top
C26  75,73.21 90 top
C28  51.3,72.31 0 top
C29  84,49.51 180 top
C30  74.6,23.31 180 top
C31  65,67.61 90 top
C33  63.6,77.91 180 top
C34  128.8,88.21 270 top
C35  125.1,77.61 0 top
C36  126.4,83.21 0 top
C37  123.9,60.21 0 top
C38  65.1,30.61 180 top
C39  51.2,54.11 0 top
C40  120.5,89.91 90 top
C41  118.1,66.61 90 top
C42  73.6,35.11 270 top
C43  42.7,49.61 90 top
C44  21.2,41.21 270 top
C45  28.8,43.41 90 top
C46  124.8,50.01 90 top
C47  87.1,41.81 180 top
C49  115.9,52.61 0 top
C50  83.6,34.11 0 top
CI  43.8,67.71 90 top
CI1  47.6,68.51 90 top
CII2  48,45.41 180 top
CII3  47.3,41.71 180 top
CII4  68.9,44.41 0 top
CII5  68.9,39.11 0 top
D1  65.3,63.81 0 top
D2  68.5,60.71 0 top
D3  69.7,10.01 90 top
I  4.4,40.01 90 top
IC2  76.2,27.01 270 top
IC3  38.6,64.71 0 top
IC5  31.4,82.31 270 top
IC6  66.1,88.21 180 top
IC7  70,70.91 270 top
IC9  102.2,79.11 90 top
IC10  88.1,81.01 90 top
IC11  34.7,36.51 270 top
IC13  OPA177S  [SO08']  66,49.01 270 top
IC14  85.7,53.21 270 top
IC15  124.3,88.21 180 top
IC16  121.9,65.11 180 top
IC17  OPA177S  [SO08']  49.9,36.51 90 top
IC18  87.1,37.81 270 top
IC19  120.9,50.01 180 top
II  4.4,32.01 90 top
IN  34.6,10.01 0 top
IN_BUF  76.6,10.01 0 top
IN_MOD  104.6,10.01 0 top
MOD_BIAS  4.4,88.01 90 top
NOISE  48.6,10.01 0 top
OUT  62.6,10.01 0 top
OUT_BUF  90.6,10.01 0 top
OUT_MOD  118,10.01 0 top
P  4.4,48.01 90 top
R1  75.1,68.81 270 top
R1*  73.8,46.81 0 top
R2  25.5,81.21 180 top
R3  40.6,59.71 0 top
R4  93.9,52.21 180 top
R5  85.1,26.01 180 top
R6  39.8,81.41 180 top
R7  65.1,72.81 90 top
R8  39.8,70.71 270 top
R9  95,83.71 270 top
R10  70,67.01 180 top
R13  65,81.51 90 top
R14  69.9,76.51 180 top
R15  54.9,38.51 90 top
R16  61,47.01 270 top
R17  75.9,43.21 180 top
R18  95.1,80.41 0 top
R19  88.1,77.31 0 top
R21  77,46.91 270 top
R22  49.9,31.11 0 top
R23  66,54.41 180 top
R24  73.3,88.21 90 top
R25  123.2,81.51 90 top
R26  33.2,64.71 270 top
R27  31.4,89.81 180 top
R32*  28.4,37.61 180 top
R32*2  28.4,33.21 180 top
R32*3  28.4,35.41 0 top
R33  61.9,71.81 180 top
R34  34.7,40.31 180 top
R35  131.5,88.21 90 top
R36  123.2,73.71 90 top
R37  119.9,72.61 180 top
R38  125.8,65.11 90 top
R39  119.9,70.11 180 top
R*  42.7,41.71 180 top
RG  36.5,80.41 90 top
RG1  34.5,74.01 0 top
RI  36.4,59.71 0 top
RI1  37.9,51.11 90 top
RII2  54.9,34.31 90 top
RII3  52.4,26.71 0 top
RII4  60.1,50.21 0 top
RII5  56.1,50.51 90 top
RP  32.7,77.51 90 top
RP1  25.3,66.61 90 top
SPST1  53.4,67.71 0 top
SPST2  24,44.91 270 top
SPST3  47.3,51.71 90 top
SPST4  69,33.01 270 top
SWITCH1  6.8,56.01 270 top
SWITCH2  6.8,24.01 270 top
SWITCH4  6.8,64.01 270 top
X7  156.5,50.01 0 top

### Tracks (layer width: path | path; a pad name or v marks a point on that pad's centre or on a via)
+10V
  Top 0.61: IC9.6 96.05,80.38 R18.2 | BIAS.3 MOD_BIAS.3
  Bottom 0.61: IC9.6 93.52,75.51 7.63,75.51 BIAS.3
+12V  (via drill 0.8 pad 1.27)
  Top 0.406: C38.1 66.2,30.61 | 66.2,30.61 SPST4.P$4 | SPST3.P$4 50.1,53.96 | 50.1,53.96 C39.1 | 66.2,30.61 66.4,30.61 v66.4,28.81 | 50.1,53.96 49.9,53.96 v49.9,55.91 | 54.3,63.06 C23.1 54.38,63.24 SPST1.P$4 | SPST2.P$4 C44.1 21.2,42.21 v19.2,42.21
  Top 0.61: C18.1 108.6,77.84 IC9.2 | IC10.7 83.1,80.38 C16.1 arc90 83.05,80.01 v81.3,80.01 | IC6.7 66.73,83.21 C15.1 67.2,83.21 v67.2,81.41 | IC15.7 124.94,83.21 125.4,83.21 | 125.4,83.21 C36.1 | 125.4,83.21 v125.4,81.41 | v122.9,58.41 122.9,60.16 C37.1 122.53,60.21 IC16.7 | v34.7,88.81 32.35,88.81 | 32.35,88.81 31.55,88.51 R27.2 | 32.35,88.81 C14.1 32.35,82.95 IC5.7 | v54.3,61.31 54.3,63.06 | C12.1 37.97,69.71 | 37.97,69.71 IC3.7 37.97,65.41 34.7,65.41 34.7,64.71 R26.2 | v37.6,71.71 37.97,71.71 37.97,69.71 | v42.9,35.41 42.9,35.46 C10.1 44.8,35.88 IC17.7 49.2,35.88 49.2,32.81 49.9,32.81 R22.2 | v72.8,50.01 72.75,50.06 C21.1 71,49.65 IC13.7 67.17,49.65 66,50.81 R23.2 | IC2.7 81.2,27.65 C25.1 83.1,28.06 v83.1,28.01 | IC14.7 88.3,53.81 90.6,53.81 C24.1 90.6,54.11 v92.5,54.11 | v136.8,11.11 136.8,10.91 | 136.8,10.91 140.1,10.91 C19.+ | v136.8,11.11 v136.8,12.71 v135.3,12.71 | v135.3,11.11 v136.8,11.11 | 136.8,10.91 135.3,10.91 135.3,11.91 | 135.3,12.41 135.3,12.91 139.2,12.91 139.2,12.41 135.3,12.41 | 135.3,12.41 135.3,11.91 | 135.3,11.91 139.1,11.91 139.1,11.41 135.4,11.41 | IC19.7 121.53,49.06 C46.1 v124.8,47.11 | IC18.7 88.05,38.45 C47.1 v90.1,41.81 | v77.2,72.31 77.15,72.26 C26.1 75.2,71.55 IC7.7 70.6,71.55 70.6,75.11 69.9,75.11 R14.2 | IC11.7 39.72,37.15 arc-90 C11.1 v39.8,35.01
  Top 1.016: X7.A26 152.1,25.88 152.1,12.51 140.1,12.51
  Top 1.422: 140.1,12.51 C19.+
  Route3 0.61: 125.2,81.21 v125.4,81.41 | v72.8,50.01 64.3,50.01
  pour Route3 (isolate 0.406): 133.7,9.81 138.7,9.81 138.7,93.51 4.3,93.51 4.3,21.51 108,21.51 108,78.31 101.8,78.31 101.8,69.61 89.2,69.61 89.2,29.41 76,29.41 76,22.61 68.1,22.61 68.1,30.91 45,30.91 45,47.31 74.2,47.31 74.2,58.71 55.6,58.71 55.6,72.21 37.3,72.21 37.3,70.51 43.3,70.51 43.3,36.81 38.1,36.81 38.1,29.31 22.9,29.31 22.9,88.41 66.1,88.41 66.1,78.91 74.2,78.91 74.2,67.41 80.2,67.41 80.2,77.31 85.2,77.31 85.2,91.91 121.7,91.91 121.7,23.41 133.7,23.41
-10V  (via drill 0.8 pad 1.27)
  Top 0.61: R19.1 87.15,81.65 IC10.6 82.97,81.65 v80.4,84.21 | BIAS.1 MOD_BIAS.1
  Bottom 0.61: v80.4,84.21 9.87,84.21 BIAS.1
-12V  (via drill 0.8 pad 1.27)  (1 unrouted)
  Top 0.406: SPST4.P$7 73.6,33.34 | 73.6,33.34 C42.2 | SPST3.P$7 44.5,51.41 42.7,51.41 | 42.7,51.41 C43.2 | SPST1.P$7 53.08,72.31 | 53.08,72.31 C28.2 | 73.6,33.34 75.5,33.34 v75.5,33.41 | 42.7,51.41 40.8,51.41 v40.8,51.31 | 53.08,72.31 53.08,74.11 v53,74.11 | C3.2 28.8,78.46 | SPST2.P$7 28.8,45.24 C45.2 30.5,44.36 v30.5,43.21
  Top 0.61: IC10.4 90.7,84.66 C1.2 v92.4,84.81 | IC6.4 62.3,90.81 C2.2 60.5,90.86 v60.5,85.71 | IC15.4 120.5,90.81 C40.2 arc-90 120.35,90.71 v118.7,90.71 | v116.3,67.61 118.1,67.61 C41.2 120,67.56 IC16.4 | v65.3,45.31 63.6,45.31 C22.2 63.38,45.31 IC13.4 | 52.52,40.21 IC17.4 | v50.8,40.21 52.45,40.21 C7.2 | IC3.4 42.45,62.11 C5.2 42.45,63.81 v42,63.81 | v28.4,76.81 28.4,78.71 C3.2 28.8,78.71 IC5.4 | IC2.4 73.6,23.36 C30.2 71.5,23.31 v71.5,24.21 | v81.2,49.51 C29.2 83.05,51.31 IC14.4 | v128.5,11.11 128.5,10.91 131.8,10.91 C20.- | v128.5,11.11 v128.5,12.71 v127,12.71 | v128.5,11.11 v127,11.11 v127,12.71 | v127,12.71 127,12.91 130.8,12.91 130.8,12.41 127,12.41 127,11.91 130.8,11.91 130.8,11.51 127,11.51 | IC19.4 C49.2 116.6,52.61 v116.6,54.41 | IC18.4 84.5,34.11 C50.2 84.55,32.21 v84.5,32.21 | v63.1,67.81 63.85,68.56 C31.2 66.95,68.56 IC7.4 | IC11.4 C6.2 32.15,32.51 v34,32.51
  Top 1.016: X7.A24 153.96,31.01 150.8,31.01 150.8,14.31 131.8,14.31 C20.-
  Route3 0.61: 53.05,74.22 v53,74.11
  pour Route3 (isolate 0.406): 113.8,9.81 130.2,9.81 130.2,15.51 119.6,15.51 119.6,90.71 86.8,90.71 86.8,75.81 81.8,75.81 81.8,65.31 72.8,65.31 72.8,77.41 64.2,77.41 64.2,87.11 25.1,87.11 25.1,31.01 36.9,31.01 36.9,38.01 42.4,38.01 42.4,69.61 35.6,69.61 35.6,73.51 58,73.51 58,60.11 75.3,60.11 75.3,46.01 46.9,46.01 46.9,32.31 69.8,32.31 69.8,24.11 74.5,24.11 74.5,31.11 87.6,31.11 87.6,71.01 99.8,71.01 99.8,79.91 113.8,79.91
BIAS_MOD_BUF_OUT  (via drill 0.8 pad 1.27)
  Top 0.61: IC19.2 121.53,50.65 120.27,49.38 IC19.6 120.27,45.45 121.8,43.91 v140,43.91
  Bottom 0.61: X7.C18 146.59,43.91 v140,43.91
DG
  Top 0.406: SPST2.P$8 33.02,45.89 35.65,43.26 R34.1
  Top 0.61: IC11.6 35.3,35.88 35.3,39.91 35.65,39.91 R34.1
DI
  Top 0.406: 52.42,70.25 SPST1.P$8 47.6,70.51
  Top 0.61: IC3.6 39.23,69.76 R8.2 43.7,69.76 | CI.2 43.7,69.76 | 43.7,69.76 47.6,69.76 47.6,70.21 47.6,70.51 CI1.2
DI_BUF_OUT  (via drill 0.8 pad 1.27)
  Top 0.61: IC18.2 86.47,38.45 87.73,37.18 IC18.6 89.73,37.21 93,37.21 99.2,31.01 v140,31.01
  Bottom 0.61: X7.C24 140.85,30.96 v140,31.01
DII1  (via drill 0.8 pad 1.27)
  Top 0.406: 44.8,50.74 SPST3.P$8 44.5,48.41 41.75,45.66 41.75,44.41 R*.2
  Top 0.61: RII5.1 57.25,44.16 59.1,46.01 59.1,50.16 RII4.1 | IC17.6 43.06,37.15 41.75,38.46 R*.2 | v43.21,44.16 41.75,44.16 41.75,44.41
  Bottom 0.61: RII5.1 v43.21,44.16
DII2
  Top 0.406: SPST4.P$8 71.8,37.21 72.9,38.31 72.9,42.51 73.6,43.21 R17.2
  Top 0.61: IC18.3 76.83,37.18 74.95,39.06 R17.2 74.75,43.41 R1*.2 | IC13.6 74.75,48.38 R1*.2 | R1*.2 74.9,46.96
ERR_BUF
  Top 0.61: IC14.3 77.53,52.58 72.31,57.8 D2.A 70.95,62.07 R10.1 70.95,70.28 IC7.6 75.1,70.28 R1.1
ERR_BUF_OUT  (via drill 0.8 pad 1.27)
  Top 0.61: IC14.2 85.06,53.85 86.33,52.58 IC14.6 90.6,52.58 v90.6,52.21 R4.2
  Bottom 0.61: OUT_BUF.1 90.6,13.71 93.4,16.51 93.4,49.41 v90.6,52.21
GND  (via drill 0.8 pad 1.27, 2.4 pad 3.81)
  Top 0.406: SPST4.P$3 64.8,32.69 v64.8,32.61 | SPST3.P$3 51.42,52.04 v51.5,52.11 | SPST1.P$3 53.73,66.21 55.8,66.21 v55.8,64.81 | SPST2.P$3 19.6,44.59 v19.6,46.11 | v26.8,42.61 28.7,42.61 C45.1
  Top 0.61: C18.2 108.6,82.92 IC9.4 106.01,84.66 R9.1 | C1.1 v86.8,84.81 | C33.2 v60.3,77.91 | C2.1 v62.3,87.11 | C40.1 v120.5,87.11 | C36.2 v129.2,83.21 | C35.2 v130.4,77.61 | C37.2 v126.7,60.21 | C41.1 v118.1,63.81 | R39.2 v116.6,70.11 | R16.2 v61,44.21 | R15.2 v54.9,41.31 | v44.8,31.71 C10.2 | v75.5,36.01 73.6,36.01 C42.1 | v50.8,42.31 52.55,42.31 C7.1 | v40.8,48.71 42.75,48.71 C43.1 | v54,54.11 C39.2 | C5.1 44.35,63.81 v44.4,63.81 | v50.3,74.11 50.3,72.31 C28.1 | v26.6,76.81 26.6,78.71 C3.1 | v24.5,79.41 24.5,81.21 R2.2 | R3.2 v43.5,59.71 | C44.2 v21.2,38.01 | v70.9,53.81 70.9,52.06 C21.2 | v65.3,43.21 63.55,43.21 C22.1 | C26.2 v75,77.31 | C16.2 81.35,78.06 v81.3,78.01 | v35.7,71.71 35.7,69.76 C12.2 | v52.4,61.31 52.35,61.36 C23.2 | C29.1 v86.8,49.51 | C24.2 v90.6,57.91 | C25.2 v81.2,31.81 81.2,34.11 C50.1 | 132.1,4.51 140.1,4.51 140.1,6.51 131.8,6.51 C20.+ 135.1,5.51 v135.1,4.81 | 143.5,5.01 v143.5,4.81 143.5,4.51 141.1,4.51 141.1,6.31 141.2,6.31 | 143.5,6.11 v143.5,6.31 143.5,6.51 141.2,6.51 | 141.2,6.31 141.2,6.51 | 141.2,6.31 141.2,5.01 143.5,5.01 | 143.5,5.01 143.5,6.11 | 143.5,6.11 141.5,6.11 141.5,5.51 143.1,5.51 | 141.2,6.51 128.4,6.51 128.4,4.51 130.9,4.51 130.9,5.01 128.7,5.01 128.7,5.51 130.6,5.51 130.6,6.01 128.8,6.01 | v28.6,86.01 30.25,86.01 C14.2 | v77.4,23.61 75.55,23.61 C30.1 | v71.2,82.91 71.2,83.21 C15.2 | v113.1,52.61 C49.1 | C46.2 v124.8,53.01 | C47.2 v84.1,41.81 | v63.1,65.81 63.95,66.66 C31.1 | v76.1,50.11 77,49.21 R21.1 | v32.1,28.41 C6.1 27.45,30.66 R32*2.2 | C11.2 v39.8,41.11 | v64.4,28.81 64.15,29.06 C38.2
  Top 1.676: C19.- C20.+
  Top 3.81: 16.25,18.26 16.25,96.76 144.75,96.76 144.75,18.26 130.9,18.26 | 130.9,18.26 v130.9,18.76 | 130.9,18.26 16.3,18.26 16.3,27.51
  other vias: 135.1,6.31 136.7,6.31 136.7,4.81 128.4,6.31 128.4,4.81 16.75,67.51 16.75,87.51 144.15,87.51 144.15,67.51 144.15,47.51 90.5,96.26 110.5,96.26 130.5,96.26 70.5,96.26 50.5,96.26 30.5,96.26 16.75,27.51 144.15,27.51 16.75,47.51 90.5,18.76 110.5,18.76 70.5,18.76 50.5,18.76 30.5,18.76
  pour Route2 (isolate 0.61): 0,100.01 0,0.01 160,0.01 160,100.01
IN_BUF_OUT  (via drill 0.8 pad 1.27)
  Top 0.61: IC2.2 75.56,27.65 76.83,26.38 IC2.6 81.8,26.38 v81.8,26.01 R5.2
  Bottom 0.61: IN_BUF.1 76.6,20.81 v81.8,26.01
ING  (via drill 0.8 pad 1.27)
  Top 0.406: SPST2.P$6 24.1,44.59 v24.1,28.01
  Bottom 0.61: SWITCH2.P$2 9.34,21.81 24.1,21.81 v24.1,28.01
INI  (via drill 0.8 pad 1.27)
  Top 0.406: SPST1.P$6 53.73,67.71 v50.5,67.71
  Bottom 0.61: v50.5,67.71 21.9,67.71 19.3,70.31 9.34,70.31 SWITCH4.P$2
INII  (via drill 0.8 pad 1.27)
  Top 0.406: v40.3,52.91 41.9,52.91 42.77,52.04 SPST3.P$6 | SPST4.P$6 68.9,32.69 68.9,26.81 60.7,26.81 60.7,37.61 v52.5,45.81
  Bottom 0.61: v52.5,45.81 45.4,52.91 v40.3,52.91 34.9,52.91 31.6,56.21 26.2,56.21 23.1,53.11 12.24,53.11 SWITCH1.P$2
N$1
  Top 0.61: R9.2 93.65,82.76 92.53,81.65 IC10.3
N$2
  cutout Route2: 28.6,38.81 33,38.81 33,41.41 38.5,41.41 38.5,34.11 30.6,34.11 30.6,32.31 28.6,32.31
  cutout Route3: 28.6,38.81 33,38.81 33,41.41 38.5,41.41 38.5,34.11 30.7,34.11 30.7,32.31 28.6,32.31
N$3
  Top 0.61: IC3.8 31.75,67.31 R26.1
N$4
  Top 0.61: R18.1 94.15,80.38 IC10.2 89,80.38 89,77.31 R19.2
N$5
  Top 0.61: R8.1 41.35,71.66 42.7,73.01 42.7,74.51 40.9,76.31 40.9,81.26 R6.1 54.9,81.41 62.85,73.46 R33.1 65.1,71.81 R7.1 65.1,71.55 IC7.2 69.4,71.55 69.4,67.51 69.05,67.51 R10.2 69.11,66.95 D1.A
N$6  (via drill 0.8 pad 1.27)
  Top 0.61: v140,41.11 103,41.11 94.8,49.31 94.8,52.16 R4.1
  Bottom 0.61: v140,41.11 140.7,41.12 X7.C20
N$7
  Top 0.61: IC16.3 121.27,70.11 R39.1
N$8  (via drill 0.8 pad 1.27)
  Top 0.61: v116.6,72.61 R37.2
  Bottom 0.61: IN_MOD.1 104.6,62.61 v116.6,72.61
N$9
  Top 0.61: IC5.2 28.84,82.91 30.3,82.91 30.8,82.41 30.8,79.31 31.65,78.46 RP.2 34.05,78.46 35,79.41 36.45,79.41 RG.1 36.4,79.36 36.4,76.61 33.8,74.01 RG1.1 26.35,74.01 RP1.2
N$10
  Top 0.61: R23.3 63.38,55.86 IC13.1
N$11
  Top 0.61: RII3.1 53,26.71 54.9,28.61 RII2.1
  Bottom 0.61: RII3.1 39,26.71 35.5,30.21 7.47,30.21 II.2
N$12
  cutout Route2: 35.3,84.71 35.3,82.31 39.8,82.31 39.8,80.21 33.8,80.21 33.8,77.61 30,77.61 30,79.91 27.6,79.91 27.6,84.71
  cutout Route3: 35.3,84.71 35.3,82.31 39.8,82.31 39.8,80.21 33.8,80.21 33.8,77.61 30,77.61 30,79.91 27.6,79.91 27.6,84.71
  cutout Route2: 73.8,73.41 73.8,70.81 76.1,70.81 76.1,68.61 71.7,68.61 71.7,66.11 68.3,66.11 68.3,68.41 66.2,68.41 66.2,73.41
  cutout Route3: 73.8,73.41 73.8,70.81 76.1,70.81 76.1,68.61 71.7,68.61 71.7,66.11 68.3,66.11 68.3,68.41 66.2,68.41 66.2,73.41
  cutout Route3: 36.1,68.51 38.7,68.51 38.7,70.21 45.5,70.21 45.5,65.01 41.1,65.01 41.1,60.91 36.1,60.91
  cutout Route2: 36.1,68.51 38.7,68.51 38.7,70.21 45.5,70.21 45.5,65.01 41.1,65.01 41.1,60.91 36.1,60.91
N$13  (via drill 0.8 pad 1.27)
  Top 0.61: R1.2 75.1,59.71 v74.2,58.81
  Bottom 0.61: D3.C 69.7,4.11 68.5,2.91 64.2,2.91 62.6,4.51 OUT.1 62.6,47.21 v74.2,58.81
N$15
  Top 0.61: C17.2 70.6,87.31 65.47,87.31 IC6.6 65.47,82.46 R13.2
N$16
  Top 0.61: R38.2 125.45,65.71 123,65.71 122.53,66.18 IC16.2 122.5,67.75 122.5,72.76 | R37.1 121,72.76 122.5,72.76 | 122.5,72.76 R36.1
N$17
  Top 0.61: IC5.3 26.4,81.68 R2.1
N$18  (1 unrouted)
  Top 0.61: 39.23,59.71 IC3.3
N$19
  Top 0.61: RP1.1 23.2,62.36 23.2,74.51 24.2,75.51 31.65,75.51 RP.1
  Bottom 0.61: RP1.1 6.65,60.26 4.4,58.01 P.2
N$20  (via drill 0.8 pad 1.27)
  Top 0.61: R38.1 125.45,64.51 121.8,64.51 121.27,63.98 IC16.6 121.27,60.18 v120.9,59.81 120.27,59.18 IC19.3
  Bottom 0.61: v120.9,59.81 118,56.91 OUT_MOD.1
N$21
  Top 0.61: R32*2.1 R32*3.2 29.35,35.88 IC11.3
N$24
  Top 0.61: IC17.3 52.56,37.15 52.6,37.11 54.9,37.11 R15.1
N$25
  Top 0.61: IC13.3 61,48.38 R16.1
N$26
  Top 0.61: IC7.3 63.87,70.28 59.7,66.11 59.7,60.31 61.5,58.51 69.7,58.51 80.7,47.51 80.7,44.81 79.1,43.21 R17.1 76.85,45.81 R21.2
N$27
  Top 0.61: R14.3 67.4,77.86 IC7.1
N$28
  Top 0.61: R14.1 72.6,77.96 IC7.8
N$29
  Top 0.61: IC3.1 31.75,62.11 R26.3
N$30
  Top 0.61: RI1.1 37.9,54.11 35.4,56.61 35.4,59.66 RI.1
  Bottom 0.61: RI1.1 5.95,44.76 4.4,43.21 I.2
N$31
  Top 0.61: IC17.1 52.52,29.66 R22.3
N$32
  Top 0.61: IC5.8 35.9,84.22 35.9,91.26 R27.1
N$33
  Top 0.406: IC5.1
  Top 0.61: IC5.1 27.2,84.21 27.2,91.26 R27.3
N$34
  Top 0.61: IC17.8 47.28,29.66 R22.1
N$37
  Top 0.61: IC5.6 36.19,81.68 RG.2 38.8,81.36 R6.2 | 38.75,81.41 R6.2 | RG1.2 38.85,76.01 R6.2
N$38  (via drill 0.8 pad 1.27)
  Top 0.61: R5.1 v139.8,26.01
  Bottom 0.61: v139.8,26.01 141.7,24.11 147.5,24.11 148.88,25.49 X7.C26
N$39
  Top 0.61: D2.C 64.59,60.71 D1.C
N$40
  Top 0.61: 45.4,42.01 45.7,41.71 CII3.2 45.4,41.71 | R*.1 45.4,41.71 | CII2.2 45.4,45.41 45.4,41.71
N$41
  Top 0.61: R34.2 34.2,40.31 34.2,37.15 IC11.2 29.35,37.15 R32*.1
N$42
  Top 0.61: R1*.1 70.3,46.81 CII4.2 70.3,40.25 CII5.2
N$43  (via drill 0.8 pad 1.27)
  Top 0.61: IC2.3 71.06,26.38 68,23.31 v34.6,23.31 32.4,23.31 25,30.71 25,34.71 25.7,35.41 R32*3.1 R32*.2
  Bottom 0.61: IN.1 v34.6,23.31
N$46
  Top 0.61: R23.1 68.62,55.86 IC13.8
N$47  (via drill 0.8 pad 1.27)
  Top 0.61: v58,60.41 58,70.81 59,71.81 R33.2
  Bottom 0.61: v58,60.41 58,33.21 47.7,22.91 47.7,15.41 48.6,14.51 NOISE.1
N$50
  Top 0.61: R24.2 73.3,89.71 C17.1 70.6,89.11 66.73,89.11 IC6.2
N$51  (via drill 0.8 pad 1.27)
  Top 0.61: v56.3,90.41 58.7,92.81 65.47,92.81 IC6.3
  Bottom 0.61: v56.3,90.41 13.53,90.41 BIAS.2
N$52
  Top 0.61: C34.2 128.8,87.31 123.67,87.31 IC15.6 123.67,82.46 R25.2
N$53
  Top 0.61: IC15.2 124.94,89.11 128.8,89.11 C34.1 131.5,89.71 R35.2
N$54  (via drill 0.8 pad 1.27)
  Top 0.61: v123.6,93.61 123.67,93.61 IC15.3
  Bottom 0.61: v123.6,93.61 8.73,93.61 MOD_BIAS.2
SG  (via drill 0.8 pad 1.27)
  Top 0.406: SPST2.P$1 v21.2,51.41
  Bottom 0.61: II.3 I.3 1.86,46.81 | 1.86,46.81 P.3 | v21.2,51.41 15.6,51.41 10.8,46.61 2.06,46.61 1.86,46.81
SI
  Top 0.406: 52.42,65.17 SPST1.P$1 51.37,65.97 CI1.1
  Top 0.61: 37.97,59.71 IC3.2 37.97,63.98 39.6,65.61 43.7,65.61 | 37.97,59.71 37.97,57.43 RI1.2 | RI.2 37.97,59.71 | CI.1 43.7,65.61 | 43.7,65.61 47.6,65.61 CI1.1
SII1
  Top 0.406: CII2.1 50.1,45.85 SPST3.P$1
  Top 0.61: RII2.2 54.9,35.88 IC17.2 50.53,35.88 49.2,37.21 49.2,41.21 CII3.1 48.7,41.91 49.2,42.41 49.2,44.07 CII2.1 | 54.9,35.36 RII2.2 | RII3.2 58.75,34.13 57,35.88 54.95,35.88 RII2.2
SII2
  Top 0.406: SPST4.P$1 66.2,39.11 CII5.1
  Top 0.61: RII5.2 58.75,56.86 61,54.61 61,50.26 RII4.2 61.05,49.65 IC13.2 65.67,49.65 67,48.31 67,44.41 CII4.1 67.5,40.25 CII5.1
V_REF
  Top 0.61: R24.1 73.3,80.21 65,80.21 | 65,80.21 R13.1 | 65,80.21 65,77.91 C33.1 R7.2
V_REF_MOD
  Top 0.61: R35.1 131.5,80.21 123.2,80.21 | 123.2,80.21 R25.1 | 123.2,80.21 123.2,77.61 | R36.2 123.2,77.61 | 123.2,77.61 C35.1

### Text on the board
tNames: summator | voltage reference | Proportional | Integrator | modulation and bias sum | General purpose controller | Proportional | - | - | Integrator | + | + | Double integrator | Double integrator | Serge Grop ULISS-ST | -12/-15V | +12/+15V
